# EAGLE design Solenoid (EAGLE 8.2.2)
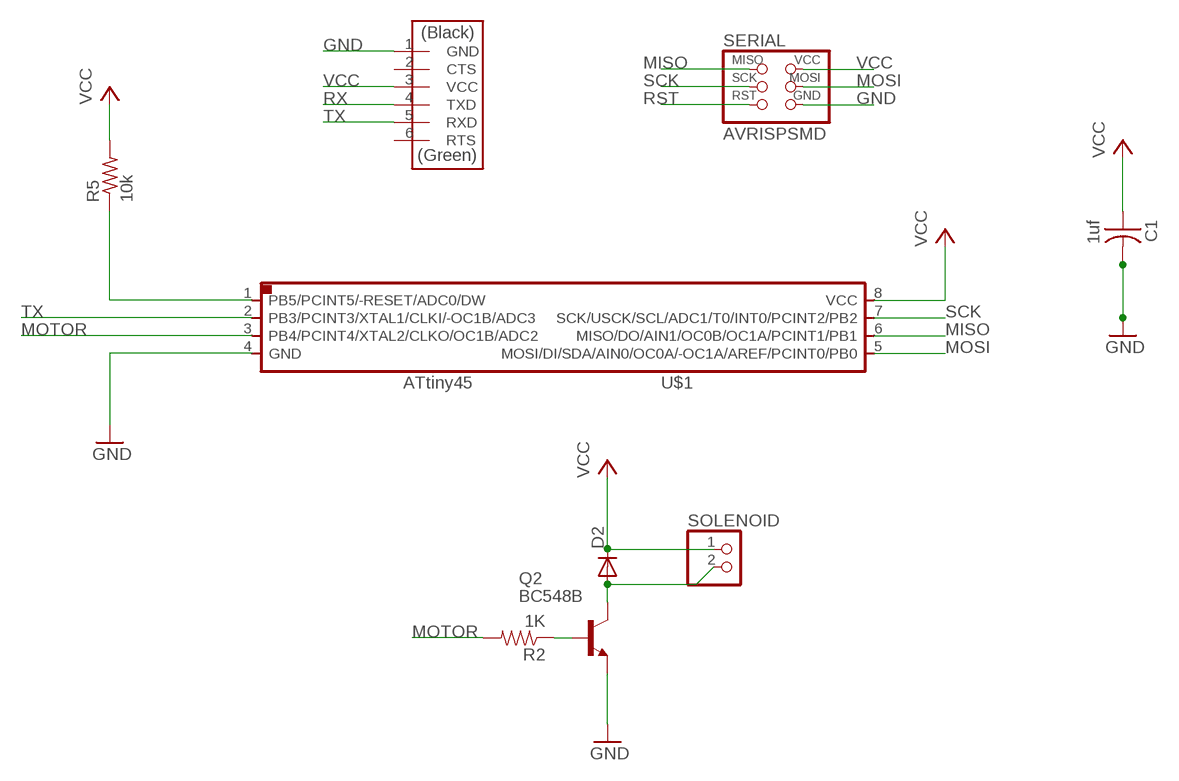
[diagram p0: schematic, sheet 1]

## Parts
C1  1uf  CAP-US1206FAB  [C1206FAB]
D2  DIODESOD123  [SOD123]
Q2  BC548B  [TO92-EBC]
R2  1K  RESISTOR1206  [1206]
R5  10k  RES-US1206FAB  [R1206FAB]
SERIAL  AVRISPSMD  [2X03SMD]
SOLENOID  PINHD-1X2  [1X02]
U$1  ATTINY45SI  [SOIC8]
U$2  FTDI-SMD-HEADER  [1X06SMD]

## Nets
GND: C1.2 Q2.E SERIAL.6(GND) U$1.4(GND) U$2.1(GND)
MISO: SERIAL.1(MISO) U$1.6(MISO/DO/AIN1/OC0B/OC1A/PCINT1/PB1)
MOSI: SERIAL.4(MOSI) U$1.5(MOSI/DI/SDA/AIN0/OC0A/-OC1A/AREF/PCINT0/PB0)
MOTOR: R2.2 U$1.3(PB4/PCINT4/XTAL2/CLKO/OC1B/ADC2)
N$3: Q2.B R2.1
N$4: D2.ANODE(A) Q2.C SOLENOID.2
RST: R5.1 SERIAL.5(RST) U$1.1(PB5/PCINT5/-RESET/ADC0/DW)
RX: U$2.4(TXD)
SCK: SERIAL.3(SCK) U$1.7(SCK/USCK/SCL/ADC1/T0/INT0/PCINT2/PB2)
TX: U$1.2(PB3/PCINT3/XTAL1/CLKI/-OC1B/ADC3) U$2.5(RXD)
VCC: C1.1 D2.CATHODE(C) R5.2 SERIAL.2(VCC) SOLENOID.1 U$1.8(VCC) U$2.3(VCC)
Unconnected: U$2.2(CTS) U$2.6(RTS)

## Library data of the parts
C1 = 01_fab_2016:CAP-US
D2 = 01-fab:DIODE: DIODE
Q2 = transistor-npn:BC548*: NPN Transistor
R2 = SparkFun-Passives:RESISTOR: Resistor
R5 = 01_fab_2016:RES-US: Resistor (US Symbol)
SERIAL = 01_fab_2016:AVRISP
SOLENOID = pinhead:PINHD-1X2: PIN HEADER
U$1 = 01-fab:ATTINY45
U$2 = 01-fab:FTDI-SMD-HEADER

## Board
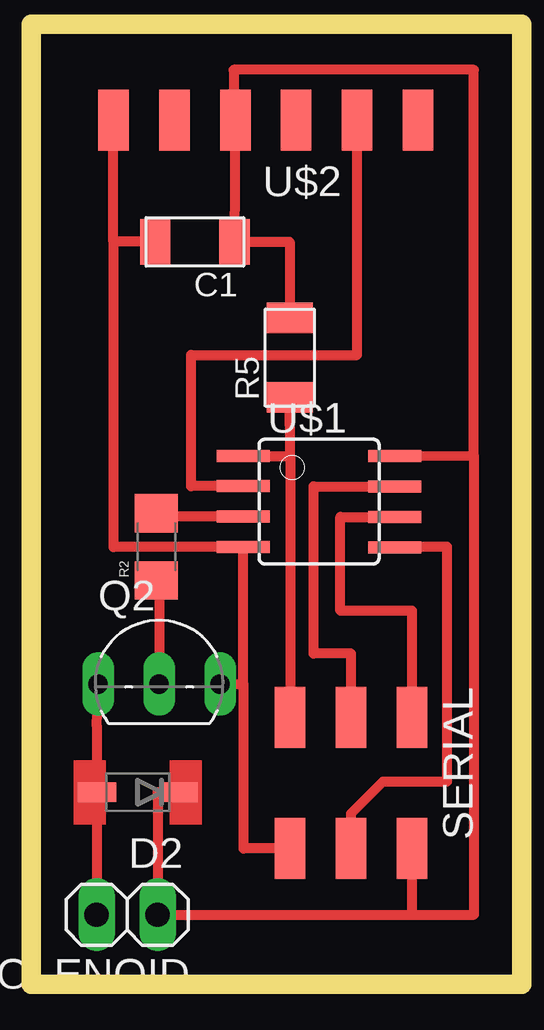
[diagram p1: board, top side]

No outline drawn. Coordinates in mm, seen from the top.
Copper layers (1*16): Top 0.035mm / dielectric 1.5mm / Bottom 0.035mm
Design rules "default *": minimum track width 10mil, minimum drill 24mil, track to track 16mil, track to pad 16mil, pad to pad 16mil, via to via 16mil, smd to smd 16mil, copper to edge 40mil, drill to drill 8mil, minimum pad ring 10mil, minimum via ring 8mil, stop-mask expansion 4mil, vias tented up to drill 0mil, thermal gap 10mil
Milling: 4 lines

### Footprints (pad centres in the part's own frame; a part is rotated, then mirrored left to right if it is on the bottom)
C1206FAB = smd 1.27 x 1.905: 1 -1.651,0; 2 1.651,0
SOD123 = smd 1.6 x 0.8: ANODE 1.7,0; CATHODE -1.7,0
TO92-EBC = drill 0.813 long: B 0,-1.27; C -2.54,-1.27; E 2.54,-1.27
1206 = smd 1.6 x 1.8: 1 -1.4,0; 2 1.4,0
R1206FAB = smd 1.27 x 1.905: 1 -1.651,0; 2 1.651,0
2X03SMD = smd 2.54 x 1.27: 1 -2.54,2.54; 2 2.92,2.54; 3 -2.54,0; 4 2.92,0; 5 -2.54,-2.54; 6 2.92,-2.54
1X02 = drill 1.016 long: 1 -1.27,0; 2 1.27,0
SOIC8 = smd 0.5 x 2.2: 1 -1.905,-3.154; 2 -0.645,-3.154; 3 0.625,-3.154; 4 1.895,-3.154; 5 1.905,3.154; 6 0.635,3.154; 7 -0.635,3.154; 8 -1.905,3.154
1X06SMD = smd 2.54 x 1.27: 1 0,6.35; 2 0,3.81; 3 0,1.27; 4 0,-1.27; 5 0,-3.81; 6 0,-6.35

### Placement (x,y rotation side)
C1  7.27,31.38 180 top
D2  4.89,8.45 180 top
Q2  5.78,14.22 0 top
R2  5.67,18.67 90 top
R5  11.22,26.56 90 top
SERIAL  13.78,9.02 270 top
SOLENOID  4.45,3.33 180 top
U$1  12.45,20.56 270 top
U$2  10.22,36.45 90 top

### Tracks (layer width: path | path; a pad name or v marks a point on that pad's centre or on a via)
GND
  Top 0.406: 3.87,31.39 3.87,18.66 U$1.4 9.29,12.95 | 3.87,31.39 U$2.1 | C1.2 3.87,31.39 | SERIAL.6 9.29,6.1 9.29,12.95 | Q2.E 9.29,12.95
MISO
  Top 0.406: SERIAL.1 16.32,16 13.34,16 13.34,19.92 U$1.6
MOSI
  Top 0.406: SERIAL.4 13.78,7.56 15.11,8.89 17.78,8.89 17.78,18.67 15.6,18.67 U$1.5
MOTOR
  Top 0.406: U$1.3 5.67,19.93 R2.2
N$3
  Top 0.406: R2.1 5.78,17.27 Q2.B
N$4
  Top 0.406: Q2.C 3.19,11.18 D2.ANODE SOLENOID.2
RST
  Top 0.406: 11.24,22.46 SERIAL.5 | 11.24,22.46 R5.1 | U$1.1 11.24,22.46
SCK
  Top 0.406: SERIAL.3 13.78,14.22 12.22,14.22 12.22,21.19 U$1.7
TX
  Top 0.406: U$1.2 7.11,21.2 7.11,26.67 14.03,26.67 U$2.5
VCC
  Top 0.406: D2.CATHODE 5.71,8.45 SOLENOID.1 16.32,3.33 | 16.32,3.33 SERIAL.2 | 16.32,3.33 18.89,3.33 18.89,22.47 | 18.89,22.47 18.89,38.56 8.89,38.56 8.89,36.45 U$2.3 C1.1 11.22,31.39 R5.2 | U$1.8 18.89,22.47
(copper drawn outside any net)
  shapes: Top area x2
